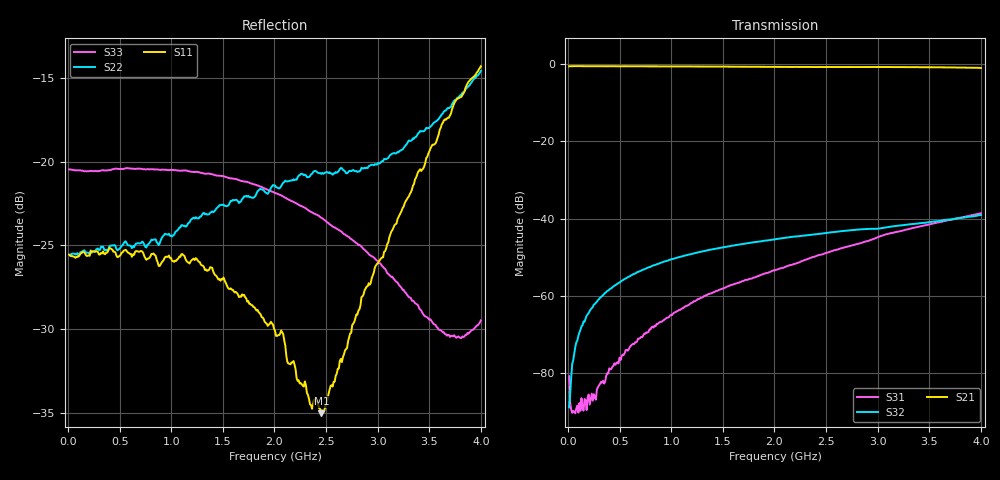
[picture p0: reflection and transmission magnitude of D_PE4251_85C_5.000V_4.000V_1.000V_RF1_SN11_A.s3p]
! Device ID: PE4251_SoldCshunt_081809
! Dir: c:\Test Bench Repositories\Bench_Software_CVI_Version_8\trunk\PSC 4Port_VNA Bench\datalog\4250\TEST\PE4251_SoldCshunt_081809\85C\5p000000\RF1
! Serial: 11
! Insertion: A
! Temp: 85C
! VDD: 5.000
! Control_Hi: 80.000
! Control_Lo: 20.000
! Logic State: RF1
! Port 1: RFC
! Port 2: RF1
! Port 3: RF2
! V1 = 1.00
! V2 = 4.00
! V3 = 1.00
! IDD: 6.328430e-05
! FILE NAME
! DATE 08/18/09  20:18
! CORRECTED  DATA
#  Hz  S  RI  R  50.00
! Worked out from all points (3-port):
!   401 points, 10 MHz to 4 GHz, reference 50 ohm
!   strongest paths, dB at 10 MHz, 1.008 GHz, 2.005 GHz, 3.002 GHz, 4 GHz:
!     S21: -0.6, -0.7, -0.8, -0.8, -1.1
!     S32: -88.8, -50.5, -45.3, -42.6, -39.0
!     S31: -80.7, -64.9, -53.3, -44.7, -38.6
!   lowest |S11| = -35.0 dB at 2.454 GHz (marker M1), VSWR 1.04, Z = 49.9 - j1.77 ohm
!   |S11| at or under -10 dB: start of sweep to end of sweep
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1e7  0.0527 0.000142  0.9305 -0.00384  -1.66e-05 -3.55e-06
     0.9301 -0.00478  0.0528 -5.27e-05  9.98e-05 5.36e-05
     2.09e-05 -8.98e-05  1.03e-05 3.5e-05  0.0947 -0.00023
9.9775e7  0.052 -0.00118  0.9322 -0.0349  2.74e-05 -2.75e-05
          0.9316 -0.0349  0.0528 -0.000983  4.31e-05 0.000298
          2.12e-05 -2.29e-05  3.47e-05 0.000304  0.0942 -0.0021
1.99525e8  0.0524 -0.00234  0.9292 -0.0689  1.04e-07 -4.62e-05
           0.9283 -0.0691  0.0533 -0.00234  6.53e-05 0.000602
           1.89e-06 -5.35e-05  5.73e-05 0.000603  0.0935 -0.00477
3.691e8  0.0532 -0.0051  0.9224 -0.1241  -5.73e-05 -6.61e-05
         0.9212 -0.1237  0.0544 -0.00456  9.8e-05 0.00112
         -5.2e-05 -7.75e-05  9.34e-05 0.00112  0.0938 -0.00943
5.287e8  0.0533 -0.00551  0.9123 -0.1758  -0.000147 -9.85e-05
         0.9119 -0.1758  0.0561 -0.00412  0.000161 0.00159
         -0.000155 -8.36e-05  0.000161 0.00159  0.0941 -0.013
1.236925e9  0.049 -0.016  0.8354 -0.3932  -0.000867 -4.67e-05
            0.8351 -0.3926  0.0651 -0.0206  0.000612 0.00356
            -0.000869 -6.63e-05  0.000603 0.00355  0.0898 -0.0251
2.005e9  0.0257 -0.0178  0.7015 -0.5838  -0.00216 0.000151
         0.7015 -0.5838  0.0716 -0.0457  0.000983 0.00532
         -0.00216 0.000151  0.000974 0.00533  0.0748 -0.0303
2.453875e9  -0.000321 -0.0177  0.6088 -0.6751  -0.00342 0.000248
            0.6074 -0.6755  0.0613 -0.0685  0.00104 0.00631
            -0.00342 0.000244  0.00104 0.00631  0.0603 -0.0315
3.650875e9  -0.1122 -0.0728  0.2816 -0.8553  -0.0089 0.00279
            0.2822 -0.8542  -0.0617 -0.1279  -0.000117 0.00958
            -0.00891 0.00276  -0.000147 0.00961  0.0053 -0.0301
4e9  -0.1762 -0.0784  0.1547 -0.873  -0.0109 0.0044
     0.1539 -0.87  -0.1372 -0.1266  -0.000744 0.0111
     -0.0109 0.00441  -0.000758 0.0111  -0.0156 -0.0298
